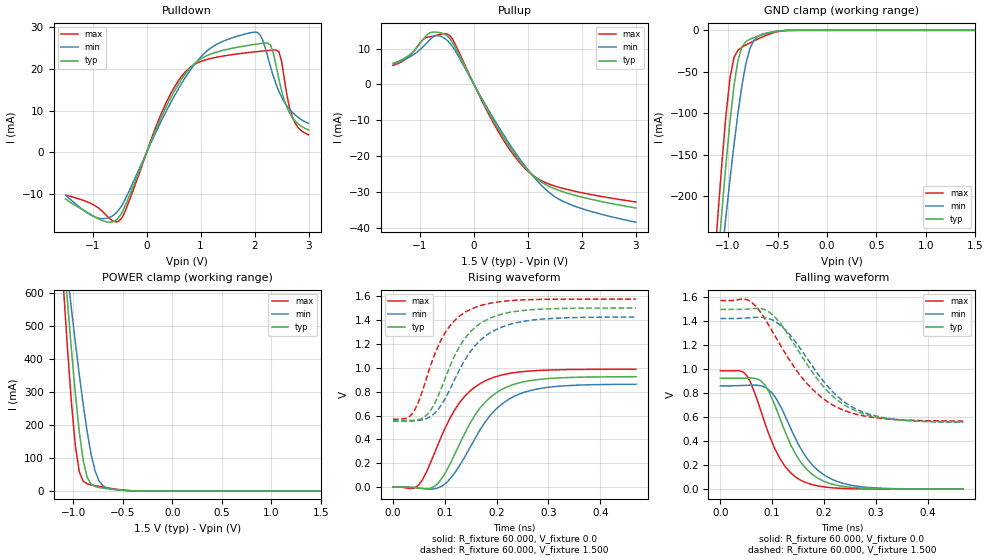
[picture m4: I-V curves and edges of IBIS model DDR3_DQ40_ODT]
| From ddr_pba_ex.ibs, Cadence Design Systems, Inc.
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|   Model DDR3_DQ40_ODT
[Model]   DDR3_DQ40_ODT
Model_type I/O
Polarity   Non-Inverting
Enable   Active-High
Vinl   =   0.575V
Vinh   =   0.925V
C_comp   1.638pF   1.631pF   1.684pF
C_comp_pullup   0.472pF   0.512pF   0.476pF
C_comp_pulldown 1.166pF   1.118pF   1.207pF
[Model Spec]
Vinh   0.925V   NA   NA
Vinl   0.575V   NA   NA
Vmeas   0.750V   NA   NA
[Add Submodel]
|  Submodel_name   Mode
DDR3_DQ_ODT60   Non-Driving
[Temperature Range]   27.000   0.125k   -40.000
[Voltage Range]   1.500V   1.425V   1.575V
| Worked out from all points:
|   slope of the pulldown table from 0 to 0.225 V, typ, clamps not added: 31.8 ohm
|   slope of the pullup table from 0 to 0.225 V, typ, clamps not added: 34.8 ohm
|   GND clamp passes 1 mA (typ) near -0.50 V on its own axis
|   POWER clamp passes 1 mA (typ) near -0.45 V on its own axis
|   rising waveform, R_fixture 60.000, V_fixture 0.0: 20-80 % time 75.7ps typ, 80.9ps min, 73.4ps max; typ from 0 V to 0.925 V
|   rising waveform, R_fixture 60.000, V_fixture 1.500: 20-80 % time 66.6ps typ, 75.2ps min, 60.6ps max; typ from 0.558 V to 1.5 V
|   falling waveform, R_fixture 60.000, V_fixture 0.0: 20-80 % time 61.5ps typ, 68.2ps min, 56.2ps max; typ from 0.926 V to 0 V
|   falling waveform, R_fixture 60.000, V_fixture 1.500: 20-80 % time 97.3ps typ, 96.9ps min, 101ps max; typ from 1.5 V to 0.56 V
[Pulldown]
|Voltage   I(typ)   I(min)   I(max)
-1.5V     -11.24mA   -10.36mA   -10.27mA
-900mV    -15.94mA   -15.8mA    -13.32mA
-500mV    -15.38mA   -13.58mA   -16.39mA
250mV     7.818mA    6.93mA     8.666mA
600mV     16.62mA    15.5mA     17.43mA
1.1V      23.14mA    24.16mA    22.24mA
1.7V      25.29mA    27.98mA    23.68mA
2.1V      26.12mA    28.29mA    24.27mA
2.3V      25.65mA    20.33mA    24.52mA
2.45V     17.59mA    14.66mA    24.19mA
2.7V      8.354mA    9.586mA    8.44mA
3V        5.378mA    6.93mA     4.234mA
[Pullup]
|Voltage   I(typ)   I(min)   I(max)
-1.5V     5.907mA    5.675mA    5.31mA
-1.2V     8.216mA    7.612mA    7.902mA
-950mV    12.44mA    10.43mA    12.49mA
-800mV    14.52mA    12.76mA    13.36mA
-650mV    14.53mA    13.64mA    13.93mA
-500mV    13.59mA    12.36mA    14.09mA
-350mV    10.47mA    9.5mA      11.3mA
450mV     -12.4mA    -11.68mA   -13.13mA
1V        -23.97mA   -23.85mA   -24.24mA
1.35V     -28.14mA   -29.63mA   -27.57mA
1.65V     -29.98mA   -32.65mA   -29.03mA
3V        -34.52mA   -38.47mA   -32.82mA
[GND_clamp]
|Voltage   I(typ)   I(min)   I(max)
-1.5V     -902.4mA   -795.2mA   -923mA
-1.14V    -333.6mA   -361.2mA   -285.4mA
-1.1V     -273.5mA   -314.1mA   -219.4mA
-1.06V    -215.4mA   -267.9mA   -157.1mA
-1.02V    -160.2mA   -222.9mA   -101.2mA
-980mV    -109.7mA   -179.4mA   -57.37mA
-940mV    -66.97mA   -138.2mA   -32.78mA
-900mV    -36.37mA   -100.2mA   -23.99mA
-820mV    -13.67mA   -40.29mA   -17.69mA
-740mV    -8.766mA   -12.21mA   -12.83mA
-540mV    -1.803mA   -1.643mA   -2.86mA
1.5V      1.911nA    275.5nA    464.3pA
[POWER_clamp]
|Voltage   I(typ)   I(min)   I(max)
-1.5V     2.395A     1.917A     2.689A
-1.1V     728.2mA    767.9mA    617.4mA
-1.06V    575.5mA    659.2mA    435.4mA
-1.02V    430.1mA    553.1mA    270.8mA
-980mV    295.8mA    450.4mA    137.9mA
-940mV    179.3mA    352.3mA    58.02mA
-900mV    91.53mA    260.8mA    29.3mA
-860mV    41.11mA    178.7mA    21.47mA
-780mV    13.3mA     60.49mA    15.94mA
-740mV    10.3mA     30.45mA    13.76mA
-620mV    5.486mA    5.676mA    7.71mA
1.5V      -5.523nA   -199nA     -1.165nA
[Ramp]
| variable   typ   min   max
dV/dt_r 0.512/74.010p   0.478/79.034p   0.547/72.510p
dV/dt_f 0.519/98.123p   0.481/97.436p   0.552/0.103n
R_load = 50.000
| The next line is not an IBIS keyword
| [Initial Delay]   0.225ns   0.350ns   0.175ns
[Rising Waveform]
R_fixture= 60.000
V_fixture= 0.0
V_fixture_min= 0.0
V_fixture_max= 0.0
|time   V(typ)   V(min)   V(max)
0s        444.9uV    1.426mV    2.714mV
49ps      -5.731mV   -6.987mV   17.22mV
65ps      -12.42mV   -14.54mV   130.8mV
83ps      17.74mV    -10.69mV   317.8mV
104ps     144.4mV    40.97mV    525.8mV
129ps     366.6mV    184.4mV    711.2mV
174ps     692.8mV    520.4mV    882mV
213ps     825.7mV    706mV      942.7mV
263ps     891.8mV    807.3mV    972.5mV
469ps     925.1mV    862mV      988.2mV
[Rising Waveform]
R_fixture= 60.000
V_fixture= 1.500
V_fixture_min= 1.425
V_fixture_max= 1.575
|time   V(typ)   V(min)   V(max)
0s        557.8mV    555.3mV    569mV
25ps      558.4mV    553.8mV    576.4mV
40ps      560.1mV    555.2mV    631.9mV
70ps      626.8mV    586.5mV    986.6mV
100ps     903.9mV    737mV      1.29V
126ps     1.16V      964.3mV    1.423V
149ps     1.299V     1.134V     1.489V
187ps     1.414V     1.292V     1.54V
242ps     1.475V     1.381V     1.567V
469ps     1.5V       1.425V     1.575V
[Falling Waveform]
R_fixture= 60.000
V_fixture= 0.0
V_fixture_min= 0.0
V_fixture_max= 0.0
|time   V(typ)   V(min)   V(max)
0s        925.6mV    862.4mV    987.7mV
45ps      926.2mV    865.7mV    974.7mV
59ps      927.8mV    868.5mV    884.7mV
79ps      900.9mV    861.9mV    641.5mV
95ps      801.8mV    822mV      442.6mV
115ps     589.6mV    699.7mV    255.2mV
155ps     226mV      340.9mV    74.62mV
190ps     87.42mV    150.2mV    25.47mV
244ps     19.35mV    40.51mV    5.087mV
469ps     222uV      223.9uV    102.7uV
[Falling Waveform]
R_fixture= 60.000
V_fixture= 1.500
V_fixture_min= 1.425
V_fixture_max= 1.575
|time   V(typ)   V(min)   V(max)
0s        1.5V       1.424V     1.574V
52ps      1.502V     1.429V     1.58V
69ps      1.509V     1.434V     1.525V
95ps      1.475V     1.421V     1.357V
129ps     1.302V     1.315V     1.108V
165ps     1.056V     1.106V     891.2mV
224ps     750.2mV    782mV      685.5mV
264ps     649.3mV    664.2mV    623mV
305ps     598.8mV    606.2mV    593.1mV
469ps     559.5mV    557.8mV    568.5mV
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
